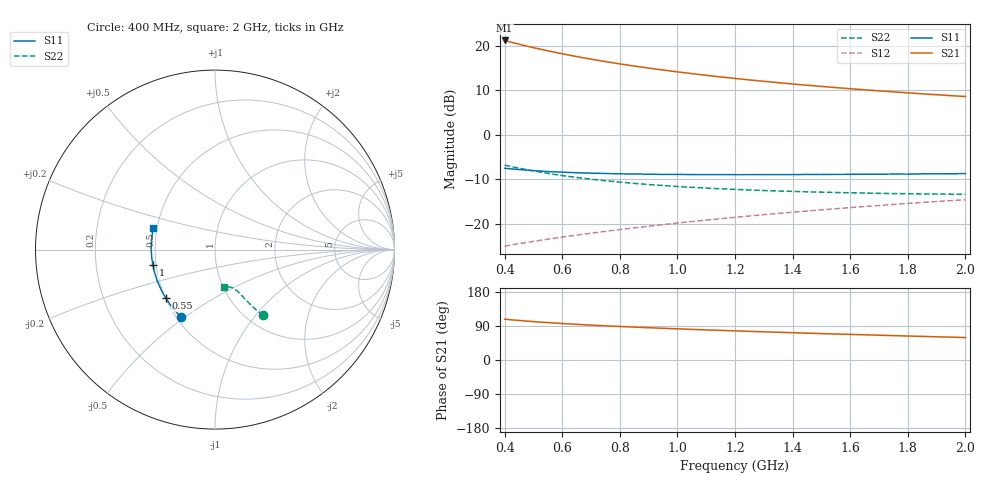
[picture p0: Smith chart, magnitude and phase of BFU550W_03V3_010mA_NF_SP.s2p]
! Filename:  P:\Prog\Test\Noise\ATS_data\Testdata_Net\06 Compressed Noise after Statistics\BFU550W_APM2013_11_D05_03p3V_010mA_NF_CM01_D.sf
! Date/Time: Tue 26/Mar/2013 16:25:27
! BFU550W_APM2013_11_D05_03p3V_1to35mA_NF_CM01_Bias6_R.sf
! Noise Parameter Data File
! BFU550W_APM2013_11_D05_03p3V_1to35mA_NF_CM01
! Date/time: Mon Mar 25 12:16:07 2013
! VAR V_out= 3.300000
! VAR I_out= 9.990000
! VAR V_in= 0.828600
! VAR I_in= 0.106210
! Device data file deembeded for feedlines and parallel
! Original file: \06 Compressed Noise after Statistics\BFU550W_APM2013_11_D05_03p3V_010mA_NF_CM01_R.sf
! Feed-files: PR019V01_070313_Feed1.s2p, PR019V01_070313_Feed2.s2p
! Parallel-file: PR019V01_070313_Par.s2p
# MHz S MA R 50
!  Freq-MHz  S11-mag  S11-arg  S21-mag  S21-arg  S12-mag  S12-arg  S22-mag  S22-arg
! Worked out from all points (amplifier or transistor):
!   37 points, 400 MHz to 2 GHz, reference 50 ohm
!   highest |S21| = 21.2 dB at 400 MHz (marker M1)
!   |S21| within 3 dB of that: start of sweep to 600.5 MHz
!   unconditionally stable (mu >= 1): 1.335 GHz to end of sweep
!   at 500 MHz: K = 0.75, MSG = 21.8 dB, |S12| = -24.0 dB
!   at 1.1 GHz: K = 0.97, MSG = 16.3 dB, |S12| = -19.2 dB
!   at 2 GHz: K = 1.02, MAG = 10.8 dB, |S12| = -14.6 dB
!   lowest NFmin = 0.71 dB at 420 MHz
!   S11 on the Smith chart (normalised r, x): 400 MHz: 0.53, -0.48; 550 MHz: 0.50, -0.32; 1 GHz: 0.48, -0.09; 2 GHz: 0.48, +0.13
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400  0.4188 -117.0  11.45 107.7  0.05573 57.8  0.4536 -53.7
420  0.4133 -119.9  11 106.3  0.05727 57.8  0.4395 -54.3
433  0.409 -121.7  10.72 105.4  0.0582 57.9  0.4306 -54.6
460  0.403 -125.1  10.19 103.7  0.06019 58.1  0.4135 -55.4
500  0.3942 -130.0  9.494 101.3  0.06307 58.4  0.3912 -56.2
550  0.3844 -135.1  8.758 98.7  0.06677 58.9  0.3669 -57.1
600  0.379 -139.9  8.108 96.2  0.07043 59.3  0.3463 -57.7
650  0.3726 -144.1  7.544 94.1  0.07421 59.8  0.3303 -58.4
700  0.369 -148.1  7.054 92.1  0.07797 60.3  0.3157 -59.0
750  0.3659 -151.6  6.623 90.2  0.08175 60.8  0.3031 -59.5
800  0.3624 -155.0  6.241 88.5  0.08563 61.2  0.293 -60.1
850  0.3609 -158.1  5.902 86.8  0.08946 61.5  0.283 -60.4
950  0.357 -163.4  5.322 83.7  0.09739 62.2  0.2678 -61.4
1000  0.3571 -166.0  5.075 82.2  0.1014 62.5  0.2611 -61.7
1100  0.355 -170.6  4.643 79.5  0.1095 62.9  0.2508 -62.9
1200  0.3546 -174.8  4.284 76.9  0.1177 63.1  0.2425 -64.2
1250  0.3547 -176.8  4.121 75.6  0.1217 63.2  0.2385 -64.6
1350  0.3551 179.7  3.839 73.2  0.1301 63.3  0.2322 -65.9
1500  0.3563 174.6  3.482 69.7  0.1427 63.1  0.2257 -68.1
1650  0.3582 169.8  3.19 66.5  0.1555 62.9  0.2204 -70.4
1750  0.3601 167.2  3.025 64.3  0.1641 62.6  0.2172 -72.0
2000  0.3649 160.5  2.682 59.3  0.1857 61.7  0.2134 -76.8
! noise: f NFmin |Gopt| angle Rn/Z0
400  0.7385  0.1012  158.5  0.0738
460  0.7215  0.1324  170.3  0.0681
600  0.7552  0.1068  163  0.0778
800  0.7816  0.1645  169.1  0.0675
1000  0.814  0.1928  172.2  0.0642
1200  0.8371  0.2209  176.9  0.0628
1400  0.8925  0.2601  -179.7  0.0548
1600  0.8831  0.2773  -176.1  0.057
1800  0.9207  0.3227  -172.8  0.0533
2000  0.9577  0.3384  -166.8  0.056
